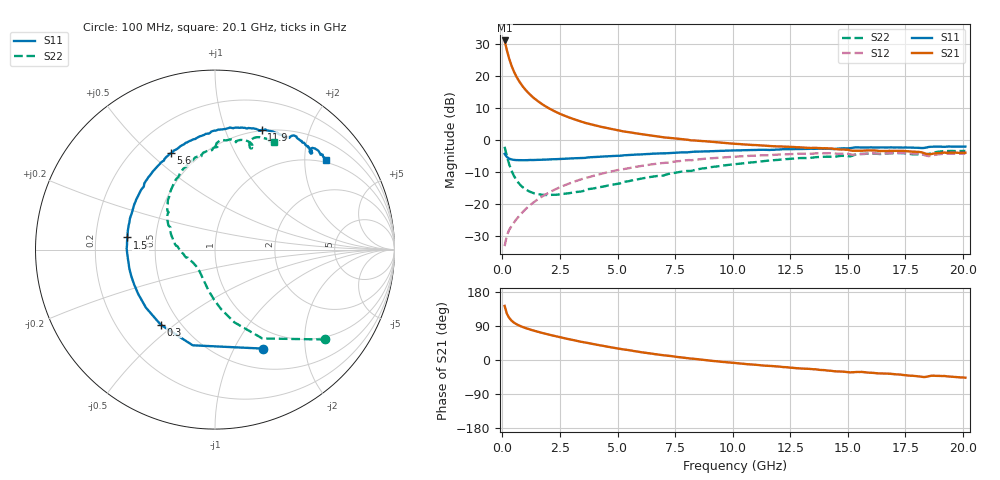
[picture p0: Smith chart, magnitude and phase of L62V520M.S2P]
!  Infineon Technologies AG
! BFR380L3 , PF131585-7, No.6, Th 09.10.01, soldered on pcb-board, measured with PP GSG850
!  Vce=2.5 V,  Ic=20.0 mA
! Common Emitter S-Parameters:  15. November 2001
#  GHz  S  MA  R  50
! f  S11  S21  S12  S22
! GHz  Mag  Ang  Mag  Ang  Mag  Ang  Mag  Ang
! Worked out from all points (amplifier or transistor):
!   201 points, 100 MHz to 20.1 GHz, reference 50 ohm
!   highest |S21| = 31.2 dB at 100 MHz (marker M1)
!   |S21| within 3 dB of that: start of sweep to 196.9 MHz
!   unconditionally stable (mu >= 1): 1.389 GHz to 4.487 GHz
!   at 3.4 GHz: K = 1.02, MAG = 8.2 dB, |S12| = -12.2 dB
!   at 10.1 GHz: K = 0.96, MSG = 2.0 dB, |S12| = -5.1 dB
!   at 20.1 GHz: K = 0.99, MSG = 0.1 dB, |S12| = -4.1 dB
!   S11 on the Smith chart (normalised r, x): 100 MHz: 0.74, -1.31; 300 MHz: 0.39, -0.45; 1.5 GHz: 0.34, +0.06; 5.6 GHz: 0.35, +0.59; 11.9 GHz: 0.49, +1.34; 20.1 GHz: 0.92, +2.53
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0.1  0.6117 -64.3  36.19 142.9  0.02219 63.0  0.7916 -39.2
0.2  0.5475 -103.1  25.34 122.0  0.03281 55.4  0.5611 -61.9
0.3  0.5162 -125.9  18.7 110.9  0.04001 53.6  0.4196 -75.1
0.4  0.5027 -140.0  14.63 103.9  0.04575 54.6  0.3342 -84.1
0.5  0.4942 -149.8  11.94 98.9  0.05143 56.4  0.28 -91.0
0.6  0.4905 -156.9  10.07 95.0  0.05775 58.0  0.2431 -96.6
0.7  0.4893 -162.6  8.71 91.9  0.06384 59.5  0.2167 -101.6
0.8  0.4888 -167.3  7.67 89.1  0.07017 60.7  0.1974 -105.9
1  0.4881 -174.6  6.188 84.5  0.08325 62.3  0.1719 -113.6
1.2  0.4922 179.5  5.189 80.5  0.09653 63.2  0.1572 -120.1
1.5  0.4928 172.1  4.192 75.2  0.1168 63.6  0.145 -128.5
1.8  0.4983 166.0  3.521 70.4  0.1375 63.2  0.1401 -135.8
2.3  0.5056 157.0  2.802 63.0  0.1711 61.4  0.1408 -146.3
2.9  0.5204 147.5  2.269 54.8  0.211 58.5  0.1492 -156.5
3.5  0.5294 138.9  1.918 47.2  0.2507 54.9  0.1605 -164.1
5.6  0.591 114.4  1.319 24.8  0.3734 41.1  0.235 168.2
6.8  0.6222 102.7  1.141 14.0  0.4351 32.7  0.2784 154.1
10.1  0.6939 78.2  0.8802 -8.0  0.5542 11.3  0.4241 124.0
11.9  0.7161 68.7  0.8024 -16.9  0.5962 0.6  0.4914 109.0
13.5  0.7344 60.9  0.7614 -24.3  0.6193 -9.2  0.5377 97.6
16.8  0.7728 48.4  0.6851 -36.2  0.6263 -25.0  0.626 77.2
20.1  0.7964 39.0  0.6395 -46.7  0.6208 -38.6  0.6824 61.2
